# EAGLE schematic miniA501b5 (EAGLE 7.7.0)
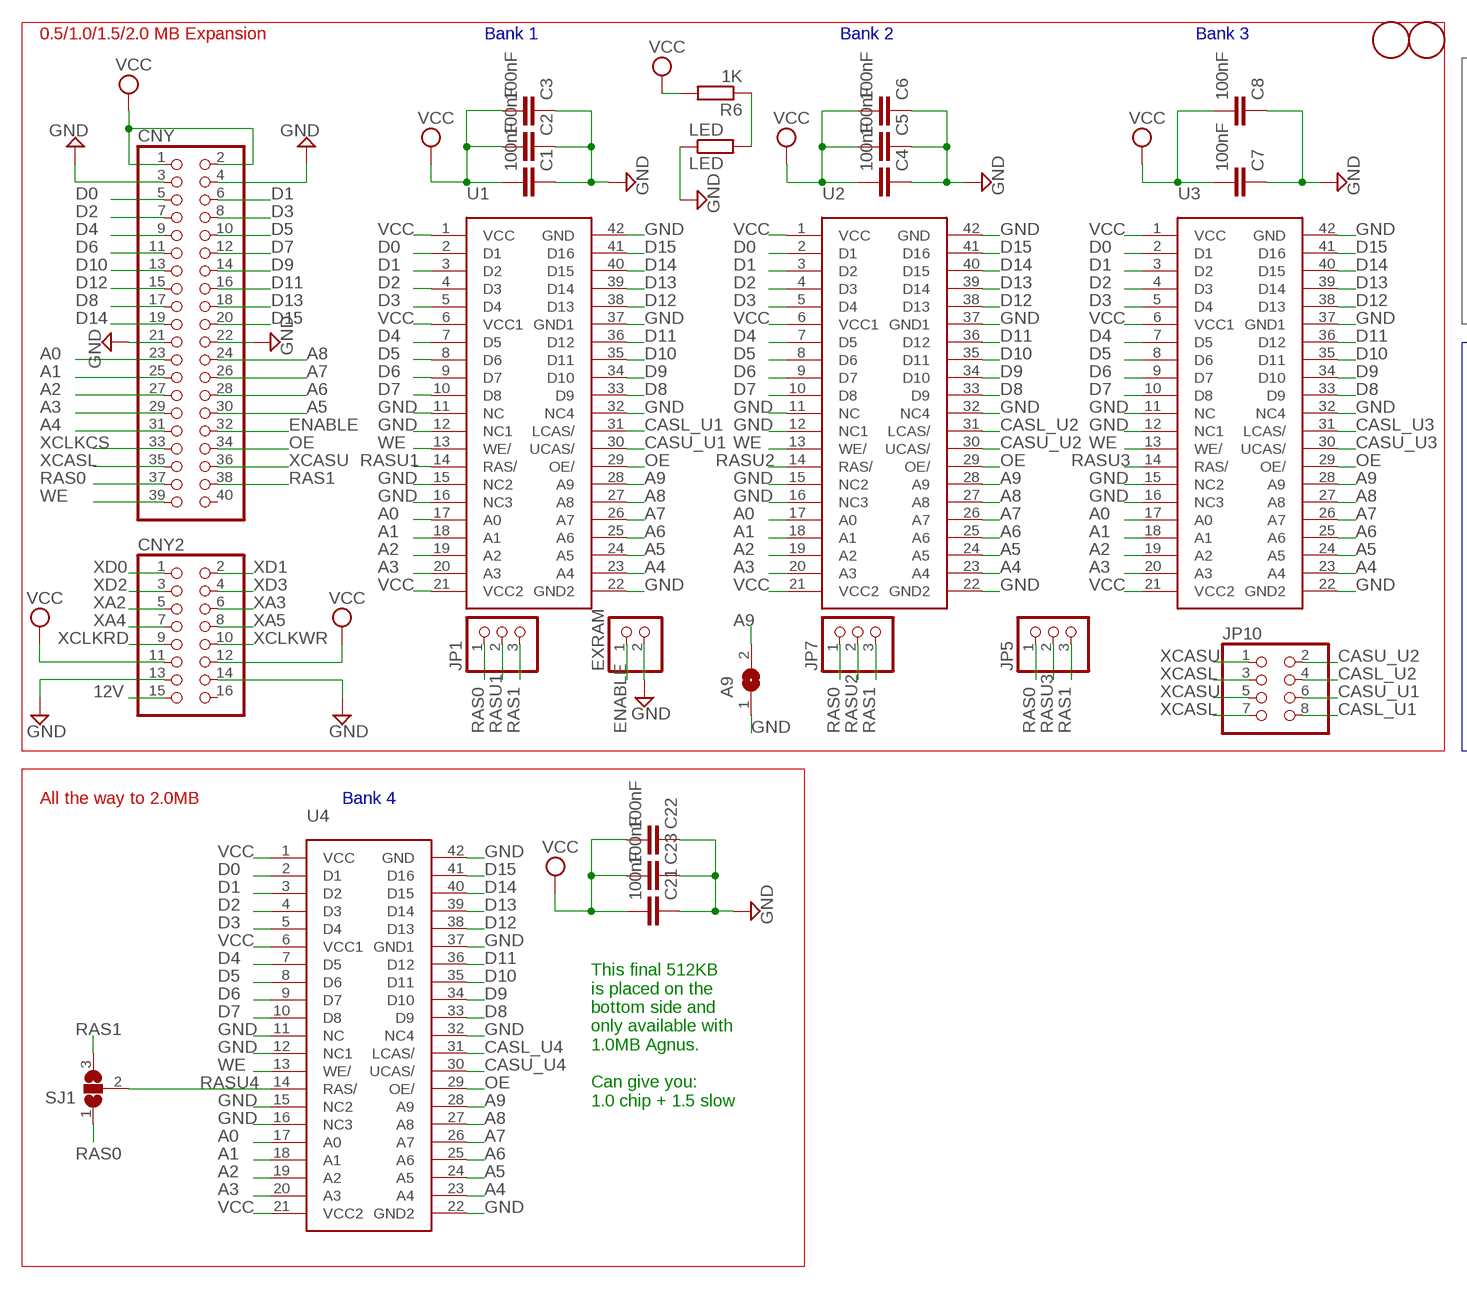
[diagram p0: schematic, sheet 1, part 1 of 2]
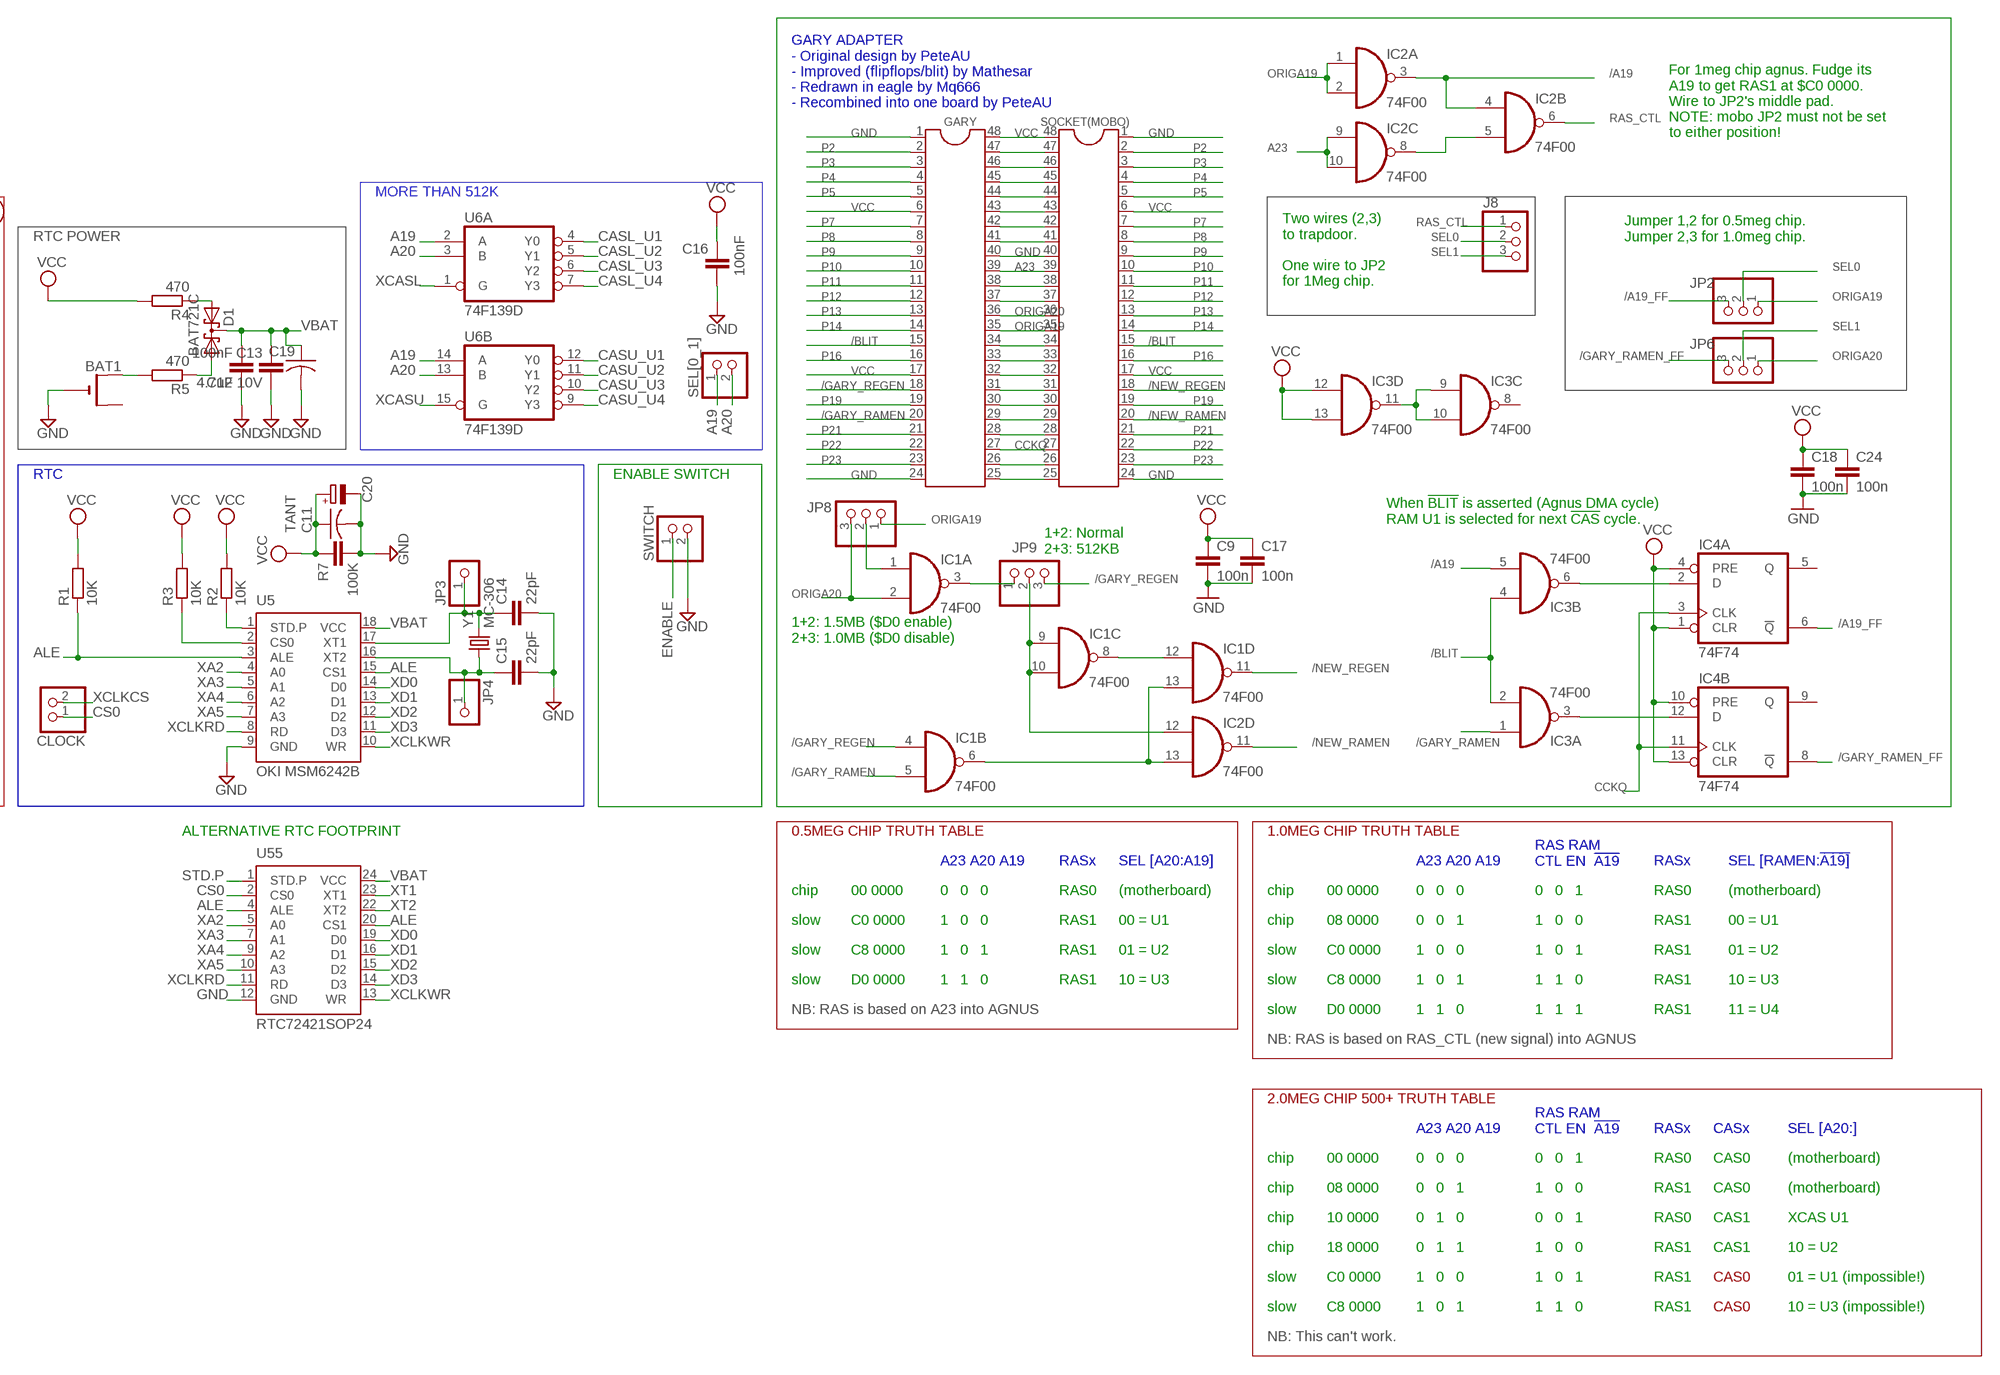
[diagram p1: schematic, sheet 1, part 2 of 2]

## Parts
A9  SJ  [SJ]
BAT1  CR2032THM  [CR2032-THRU]
C1  100nF  C-EUC0805KPZ  [C0805KPZ]
C2  100nF  C-EUC0805KPZ  [C0805KPZ]
C3  100nF  C-EUC0805KPZ  [C0805KPZ]
C4  100nF  C-EUC0805KPZ  [C0805KPZ]
C5  100nF  C-EUC0805KPZ  [C0805KPZ]
C6  100nF  C-EUC0805KPZ  [C0805KPZ]
C7  100nF  C-EUC0805KPZ  [C0805KPZ]
C8  100nF  C-EUC0805KPZ  [C0805KPZ]
C9  100n  C-EUC0805K  [C0805K]
C11  TANT  C-USC1206PZ  [C1206PZ]
C12  100nF  C-EUC0805KPZ  [C0805KPZ]
C13  4.7uF 10V  C-EUC0805KPZ  [C0805KPZ]
C14  22pF  C-EUC0805KPZ  [C0805KPZ]
C15  22pF  C-EUC0805KPZ  [C0805KPZ]
C16  100nF  C-EUC0805KPZ  [C0805KPZ]
C17  100n  C-EUC0805K  [C0805K]
C18  100n  C-EUC0805K  [C0805K]
C19  C-USC1206PZ  [C1206PZ]
C20  CPOL-EUE2.5-5  [E2,5-5]
C21  100nF  C-EUC0805KPZ  [C0805KPZ]
C22  100nF  C-EUC0805KPZ  [C0805KPZ]
C23  100nF  C-EUC0805KPZ  [C0805KPZ]
C24  100n  C-EUC0805K  [C0805K]
CLOCK  PINHD-1X2  [1X02]
CNY  PINHD-2X20  [2X20]
CNY2  PINHD-2X8  [2X08]
D1  BAT721C  BAT54C  [SOT23]
EXRAM  PINHD-1X2  [1X02]
GARY  DIL48  [DIL48]
IC1  74F00  74HCT00D  [SO14]
IC2  74F00  74HCT00D  [SO14]
IC3  74F00  74HCT00D  [SO14]
IC4  74F74  74HCT74D  [SO14]
J8  PINHD-1X3  [1X03]
JP1  PINHD-1X3  [1X03]
JP2  PINHD-1X3  [1X03]
JP3  PINHD-1X1  [1X01]
JP4  PINHD-1X1  [1X01]
JP5  PINHD-1X3  [1X03]
JP6  PINHD-1X3  [1X03]
JP7  PINHD-1X3  [1X03]
JP8  PINHD-1X3  [1X03]
JP9  PINHD-1X3  [1X03]
JP10  PINHD-2X4  [2X04]
LED  LED  R-EU_M0805PZ  [M0805PZ]
R1  10K  R-EU_M0805PZ  [M0805PZ]
R2  10K  R-EU_M0805PZ  [M0805PZ]
R3  10K  R-EU_M0805PZ  [M0805PZ]
R4  470  R-EU_M0805PZ  [M0805PZ]
R5  470  R-EU_M0805PZ  [M0805PZ]
R6  1K  R-EU_M0805PZ  [M0805PZ]
R7  100K  C-EUC0805KPZ  [C0805KPZ]
SEL[0_1]  PINHD-1X2  [1X02]
SJ1  SJ2W  [SJ_2]
SOCKET(MOBO)  DIL48  [DIL48]
SWITCH  PINHD-1X2  [1X02]
U1  DRAMSOJ40A  [SOJ40]
U2  DRAMSOJ40A  [SOJ40]
U3  DRAMSOJ40A  [SOJ40]
U4  DRAMSOJ40A  [SOJ40]
U5  OKI MSM6242B  RTC72421  [DIL18]
U6  74F139D  74LS139D  [SO16]
U55  RTC72421SOP24  [SOP24]
U$1  FIDUCIAL  [FIDUCIAL_1MM]
U$2  FIDUCIAL  [FIDUCIAL_1MM]
Y1  MC-306  [MC-306]

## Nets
12V: CNY2.15
/A19: IC2.3(A:O) IC2.4(B:I0) IC3.5(B:I1)
/A19_FF: IC4.6(A:!Q) JP2.3
/BLIT: GARY.15 IC3.2(A:I1) IC3.4(B:I0) SOCKET(MOBO).15
/GARY_RAMEN: GARY.20 IC1.5(B:I1) IC3.1(A:I0)
/GARY_RAMEN_FF: IC4.8(B:!Q) JP6.3
/GARY_REGEN: GARY.18 IC1.4(B:I0) JP9.3
/NEW_RAMEN: IC2.11(D:O) SOCKET(MOBO).20
/NEW_REGEN: IC1.11(D:O) SOCKET(MOBO).18
A0: CNY.23 U1.17(A0) U2.17(A0) U3.17(A0) U4.17(A0)
A1: CNY.25 U1.18(A1) U2.18(A1) U3.18(A1) U4.18(A1)
A2: CNY.27 U1.19(A2) U2.19(A2) U3.19(A2) U4.19(A2)
A3: CNY.29 U1.20(A3) U2.20(A3) U3.20(A3) U4.20(A3)
A4: CNY.31 U1.23(A4) U2.23(A4) U3.23(A4) U4.23(A4)
A5: CNY.30 U1.24(A5) U2.24(A5) U3.24(A5) U4.24(A5)
A6: CNY.28 U1.25(A6) U2.25(A6) U3.25(A6) U4.25(A6)
A7: CNY.26 U1.26(A7) U2.26(A7) U3.26(A7) U4.26(A7)
A8: CNY.24 U1.27(A8) U2.27(A8) U3.27(A8) U4.27(A8)
A9: A9.2 U1.28(A9) U2.28(A9) U3.28(A9) U4.28(A9)
A19: SEL[0_1].1 U6.2(A:A) U6.14(B:A)
A20: SEL[0_1].2 U6.3(A:B) U6.13(B:B)
A23: GARY.39 IC2.9(C:I0) IC2.10(C:I1) SOCKET(MOBO).39
ALE: R1.P$1 U5.3(ALE) U5.15(CS1) U55.4(ALE) U55.20(CS1)
CASL_U1: JP10.8 U1.31(LCAS/) U6.4(A:Y0)
CASL_U2: JP10.4 U2.31(LCAS/) U6.5(A:Y1)
CASL_U3: U3.31(LCAS/) U6.6(A:Y2)
CASL_U4: U4.31(LCAS/) U6.7(A:Y3)
CASU_U1: JP10.6 U1.30(UCAS/) U6.12(B:Y0)
CASU_U2: JP10.2 U2.30(UCAS/) U6.11(B:Y1)
CASU_U3: U3.30(UCAS/) U6.10(B:Y2)
CASU_U4: U4.30(UCAS/) U6.9(B:Y3)
CCKQ: GARY.27 IC4.3(A:CLK) IC4.11(B:CLK) SOCKET(MOBO).27
CS0: CLOCK.1 R3.P$1 U5.2(CS0) U55.2(CS0)
D0: CNY.5 U1.2(D1) U2.2(D1) U3.2(D1) U4.2(D1)
D1: CNY.6 U1.3(D2) U2.3(D2) U3.3(D2) U4.3(D2)
D2: CNY.7 U1.4(D3) U2.4(D3) U3.4(D3) U4.4(D3)
D3: CNY.8 U1.5(D4) U2.5(D4) U3.5(D4) U4.5(D4)
D4: CNY.9 U1.7(D5) U2.7(D5) U3.7(D5) U4.7(D5)
D5: CNY.10 U1.8(D6) U2.8(D6) U3.8(D6) U4.8(D6)
D6: CNY.11 U1.9(D7) U2.9(D7) U3.9(D7) U4.9(D7)
D7: CNY.12 U1.10(D8) U2.10(D8) U3.10(D8) U4.10(D8)
D8: CNY.17 U1.33(D9) U2.33(D9) U3.33(D9) U4.33(D9)
D9: CNY.14 U1.34(D10) U2.34(D10) U3.34(D10) U4.34(D10)
D10: CNY.13 U1.35(D11) U2.35(D11) U3.35(D11) U4.35(D11)
D11: CNY.16 U1.36(D12) U2.36(D12) U3.36(D12) U4.36(D12)
D12: CNY.15 U1.38(D13) U2.38(D13) U3.38(D13) U4.38(D13)
D13: CNY.18 U1.39(D14) U2.39(D14) U3.39(D14) U4.39(D14)
D14: CNY.19 U1.40(D15) U2.40(D15) U3.40(D15) U4.40(D15)
D15: CNY.20 U1.41(D16) U2.41(D16) U3.41(D16) U4.41(D16)
ENABLE: CNY.32 EXRAM.1 SWITCH.1
GND: A9.1 BAT1.- C1.P$1 C2.P$1 C3.P$1 C4.P$1 C5.P$1 C6.P$1 C7.P$1 C8.P$1 C9.2 C11.P$2 C12.P$1 C13.P$2 C14.P$2 C15.P$2 C16.P$2 C17.2 C18.2 C19.P$2 C20.- C21.P$1 C22.P$1 C23.P$1 C24.2 CNY2.13 CNY2.14 CNY.3 CNY.4 CNY.21 CNY.22 EXRAM.2 GARY.1 GARY.24 GARY.40 LED.P$1 R7.P$2 SOCKET(MOBO).1 SOCKET(MOBO).24 SOCKET(MOBO).40 SWITCH.2 U1.11(NC) U1.12(NC1) U1.15(NC2) U1.16(NC3) U1.22(GND2) U1.32(NC4) U1.37(GND1) U1.42(GND) U2.11(NC) U2.12(NC1) U2.15(NC2) U2.16(NC3) U2.22(GND2) U2.32(NC4) U2.37(GND1) U2.42(GND) U3.11(NC) U3.12(NC1) U3.15(NC2) U3.16(NC3) U3.22(GND2) U3.32(NC4) U3.37(GND1) U3.42(GND) U4.11(NC) U4.12(NC1) U4.15(NC2) U4.16(NC3) U4.22(GND2) U4.32(NC4) U4.37(GND1) U4.42(GND) U5.9(GND) U55.12(GND)
N$1: LED.P$2 R6.P$1
N$2: GARY.47 SOCKET(MOBO).47
N$3: GARY.46 SOCKET(MOBO).46
N$4: GARY.45 SOCKET(MOBO).45
N$5: IC1.3(A:O) JP9.1
N$6: GARY.43 SOCKET(MOBO).43
N$7: GARY.42 SOCKET(MOBO).42
N$11: BAT1.+ R5.P$2
N$12: D1.2(A2) R4.P$1
N$14: GARY.44 SOCKET(MOBO).44
N$15: GARY.34 SOCKET(MOBO).34
N$16: D1.1(A1) R5.P$1
N$17: GARY.32 SOCKET(MOBO).32
N$18: GARY.31 SOCKET(MOBO).31
N$19: GARY.30 SOCKET(MOBO).30
N$20: GARY.29 SOCKET(MOBO).29
N$21: GARY.28 SOCKET(MOBO).28
N$23: GARY.26 SOCKET(MOBO).26
N$24: GARY.25 SOCKET(MOBO).25
N$25: IC3.6(B:O) IC4.2(A:D)
N$26: IC3.9(C:I0) IC3.10(C:I1) IC3.11(D:O)
N$27: IC3.3(A:O) IC4.12(B:D)
N$28: IC1.1(A:I0) JP8.2
N$29: IC1.9(C:I0) IC1.10(C:I1) IC2.12(D:I0) JP9.2
N$30: IC1.8(C:O) IC1.12(D:I0)
N$31: IC1.6(B:O) IC1.13(D:I1) IC2.13(D:I1)
OE: CNY.34 U1.29(OE/) U2.29(OE/) U3.29(OE/) U4.29(OE/)
ORIGA19: GARY.35 IC2.1(A:I0) IC2.2(A:I1) JP2.1 JP8.1 SOCKET(MOBO).35
ORIGA20: GARY.36 IC1.2(A:I1) JP6.1 JP8.3 SOCKET(MOBO).36
ORIGN$5: GARY.41 SOCKET(MOBO).41
ORIGN$9: GARY.38 SOCKET(MOBO).38
ORIGN$10: GARY.37 SOCKET(MOBO).37
ORIGN$13: GARY.33 SOCKET(MOBO).33
ORIGN$22: IC2.5(B:I1) IC2.8(C:O)
P2: GARY.2 SOCKET(MOBO).2
P3: GARY.3 SOCKET(MOBO).3
P4: GARY.4 SOCKET(MOBO).4
P5: GARY.5 SOCKET(MOBO).5
P7: GARY.7 SOCKET(MOBO).7
P8: GARY.8 SOCKET(MOBO).8
P9: GARY.9 SOCKET(MOBO).9
P10: GARY.10 SOCKET(MOBO).10
P11: GARY.11 SOCKET(MOBO).11
P12: GARY.12 SOCKET(MOBO).12
P13: GARY.13 SOCKET(MOBO).13
P14: GARY.14 SOCKET(MOBO).14
P16: GARY.16 SOCKET(MOBO).16
P19: GARY.19 SOCKET(MOBO).19
P21: GARY.21 SOCKET(MOBO).21
P22: GARY.22 SOCKET(MOBO).22
P23: GARY.23 SOCKET(MOBO).23
RAS0: CNY.37 JP1.1 JP5.1 JP7.1 SJ1.1
RAS1: CNY.38 JP1.3 JP5.3 JP7.3 SJ1.3
RAS_CTL: IC2.6(B:O) J8.1
RASU1: JP1.2 U1.14(RAS/)
RASU2: JP7.2 U2.14(RAS/)
RASU3: JP5.2 U3.14(RAS/)
RASU4: SJ1.2 U4.14(RAS/)
SEL0: J8.2 JP2.2
SEL1: J8.3 JP6.2
STD.P: R2.P$1 U5.1(STD.P) U55.1(STD.P)
VBAT: C12.P$2 C13.P$1 C19.P$1 D1.3(CC) U5.18(VCC) U55.24(VCC)
VCC: C1.P$2 C2.P$2 C3.P$2 C4.P$2 C5.P$2 C6.P$2 C7.P$2 C8.P$2 C9.1 C11.P$1 C16.P$1 C17.1 C18.1 C20.+ C21.P$2 C22.P$2 C23.P$2 C24.1 CNY2.11 CNY2.12 CNY.1 CNY.2 GARY.6 GARY.17 GARY.48 IC3.12(D:I0) IC3.13(D:I1) IC4.1(A:CLR) IC4.4(A:PRE) IC4.10(B:PRE) IC4.13(B:CLR) R1.P$2 R2.P$2 R3.P$2 R4.P$2 R6.P$2 R7.P$1 SOCKET(MOBO).6 SOCKET(MOBO).17 SOCKET(MOBO).48 U1.1(VCC) U1.6(VCC1) U1.21(VCC2) U2.1(VCC) U2.6(VCC1) U2.21(VCC2) U3.1(VCC) U3.6(VCC1) U3.21(VCC2) U4.1(VCC) U4.6(VCC1) U4.21(VCC2)
WE: CNY.39 U1.13(WE/) U2.13(WE/) U3.13(WE/) U4.13(WE/)
XA2: CNY2.5 U5.4(A0) U55.5(A0)
XA3: CNY2.6 U5.5(A1) U55.7(A1)
XA4: CNY2.7 U5.6(A2) U55.9(A2)
XA5: CNY2.8 U5.7(A3) U55.10(A3)
XCASL: CNY.35 JP10.3 JP10.7 U6.1(A:G)
XCASU: CNY.36 JP10.1 JP10.5 U6.15(B:G)
XCLKCS: CLOCK.2 CNY.33
XCLKRD: CNY2.9 U5.8(RD) U55.11(RD)
XCLKWR: CNY2.10 U5.10(WR) U55.13(WR)
XD0: CNY2.1 U5.14(D0) U55.19(D0)
XD1: CNY2.2 U5.13(D1) U55.16(D1)
XD2: CNY2.3 U5.12(D2) U55.15(D2)
XD3: CNY2.4 U5.11(D3) U55.14(D3)
XT1: C14.P$1 JP3.1 U5.17(XT1) U55.23(XT1) Y1.4
XT2: C15.P$1 JP4.1 U5.16(XT2) U55.22(XT2) Y1.1
Unconnected: BAT1.+2(+1) CNY2.16 CNY.40 IC3.8(C:O) IC4.5(A:Q) IC4.9(B:Q)

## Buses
B$1

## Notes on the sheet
- GARY ADAPTER
  - Original design by PeteAU
  - Improved (flipflops/blit) by Mathesar
  - Redrawn in eagle by Mq666
  - Recombined into one board by PeteAU
- For 1meg chip agnus. Fudge its
  A19 to get RAS1 at $C0 0000.
  Wire to JP2's middle pad.
  NOTE: mobo JP2 must not be set
  to either position!
- MORE THAN 512K
- 0.5/1.0/1.5/2.0 MB Expansion | Bank 1 | Bank 2 | Bank 3
- RTC POWER
- Jumper 1,2 for 0.5meg chip.
  Jumper 2,3 for 1.0meg chip.
- Two wires (2,3)
  to trapdoor.
  
  One wire to JP2
  for 1Meg chip.
- RTC | ENABLE SWITCH
- When !BLIT! is asserted (Agnus DMA cycle)
  RAM U1 is selected for next !CAS! cycle.
- 1+2: Normal
  2+3: 512KB
- 1+2: 1.5MB ($D0 enable)
  2+3: 1.0MB ($D0 disable)
- ALTERNATIVE RTC FOOTPRINT | 0.5MEG CHIP TRUTH TABLE | 1.0MEG CHIP TRUTH TABLE
- All the way to 2.0MB | Bank 4
- A23 A20 A19 | RASx | SEL [A20:A19] | A23 A20 A19
- RAS RAM
  CTL EN  !A19
- RASx | SEL [RAMEN:!A19]
- chip | 00 0000 | 0   0   0 | RAS0 | (motherboard) | chip | 00 0000 | 0   0   0 | 0   0   1 | RAS0 | (motherboard)
- slow | C0 0000 | 1   0   0 | RAS1 | 00 = U1 | chip | 08 0000 | 0   0   1 | 1   0   0 | RAS1 | 00 = U1
- slow | C8 0000 | 1   0   1 | RAS1 | 01 = U2 | slow | C0 0000 | 1   0   0 | 1   0   1 | RAS1 | 01 = U2
- slow | D0 0000 | 1   1   0 | RAS1 | 10 = U3 | slow | C8 0000 | 1   0   1 | 1   1   0 | RAS1 | 10 = U3
- NB: RAS is based on A23 into AGNUS | slow | D0 0000 | 1   1   0 | 1   1   1 | RAS1 | 11 = U4
- NB: RAS is based on RAS_CTL (new signal) into AGNUS
- This final 512KB
  is placed on the
  bottom side and
  only available with
  1.0MB Agnus.
  
  Can give you:
  1.0 chip + 1.5 slow
- 2.0MEG CHIP 500+ TRUTH TABLE
- A23 A20 A19
- RAS RAM
  CTL EN  !A19
- RASx | CASx | SEL [A20:]
- chip | 00 0000 | 0   0   0 | 0   0   1 | RAS0 | CAS0 | (motherboard)
- chip | 08 0000 | 0   0   1 | 1   0   0 | RAS1 | CAS0 | (motherboard)
- chip | 10 0000 | 0   1   0 | 0   0   1 | RAS0 | CAS1 | XCAS U1
- chip | 18 0000 | 0   1   1 | 1   0   0 | RAS1 | CAS1 | 10 = U2
- slow | C0 0000 | 1   0   0 | 1   0   1 | RAS1 | CAS0 | 01 = U1 (impossible!)
- slow | C8 0000 | 1   0   1 | 1   1   0 | RAS1 | CAS0 | 10 = U3 (impossible!)
- NB: This can't work.

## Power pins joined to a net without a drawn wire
GND: IC1.7(P:GND) IC2.7(P:GND) IC3.7(P:GND) IC4.7(P:GND) U6.8(P:GND)
VCC: IC1.14(P:VCC) IC2.14(P:VCC) IC3.14(P:VCC) IC4.14(P:VCC) U6.16(P:VCC)

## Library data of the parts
A9 = jumper:SJ: SMD solder JUMPER
BAT1 = adafruit:CR2032
C1-C8 C12-C16 C21-C23 R7 = resistorpz:C-EU: CAPACITOR, European symbol
C9 C17 C18 C24 = rcl:C-EU: CAPACITOR, European symbol
C11 C19 = resistorpz:C-US: CAPACITOR, American symbol
C20 = resistor:CPOL-EU: POLARIZED CAPACITOR, European symbol
CLOCK EXRAM SEL[0_1] SWITCH = pinhead:PINHD-1X2: PIN HEADER
CNY = pinhead:PINHD-2X20: PIN HEADER
CNY2 = pinhead:PINHD-2X8: PIN HEADER
D1 = diode:BAT54C: Schottky Diodes Source: Fairchild .. BAT54.pdf
GARY = ic-package:DIL48: Dual In Line
IC1-IC3 = 74xx-eu-mq:74*00: Quad 2-input NAND gate
IC4 = 74xx-eu-mq:74*74: Dual D type positive edge triggered FLIP FLOP, preset and clear
J8 JP1 JP2 JP5-JP9 = pinhead:PINHD-1X3: PIN HEADER
JP3 JP4 = pinhead:PINHD-1X1: PIN HEADER
JP10 = pinhead:PINHD-2X4: PIN HEADER
LED R1-R6 = resistorpz:R-EU_: RESISTOR, European symbol
SJ1 = jumper:SJ2W: SMD solder JUMPER
SOCKET(MOBO) = ic-package-nosilk:DIL48: Dual In Line
U1-U4 = memory-soj42:DRAMSOJ40A: MEMORY; OC_FARNELL: unknown; OC_NEWARK: unknown
U5 = fox-electronics:RTC72421: Real Time Clock http://www.foxonline.com/72421.htm; MPN: RTC72421B; OC_FARNELL: 1216228; OC_NEWARK: 01M8738
U6 = 74xx-us:74*139: Dual 2-line to 4-line DECODER/DEMULTIPLEXER
U55 = fox-electronics:RTC72421: Real Time Clock http://www.foxonline.com/72421.htm
U$1 U$2 = adafruit:FIDUCIAL: For use by pick and place machines to calibrate the vision/machine, 1mm
Y1 = crystal:MC-306: kHz RANGE CRYSTAL UNIT SMD; MPN: MC-306 60.0KHZ 100PPM ,12.5PF; OC_FARNELL: 1278040; OC_NEWARK: 31M5576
